DATA_BLOCK DB 49
TITLE =
VERSION : 0.1


  STRUCT
   Leiding : ARRAY  [0 .. 100 ] OF //Drukwaarde
   REAL  := 0.000000e+000;
  END_STRUCT ;
BEGIN
   Leiding[0] := 	1.138932E+00	;
Leiding[1] := 	1.155988E+00	;
Leiding[2] := 	1.173205E+00	;
Leiding[3] := 	1.190583E+00	;
Leiding[4] := 	1.208122E+00	;
Leiding[5] := 	1.225822E+00	;
Leiding[6] := 	1.243683E+00	;
Leiding[7] := 	1.261705E+00	;
Leiding[8] := 	1.279888E+00	;
Leiding[9] := 	1.298232E+00	;
Leiding[10] := 	1.316737E+00	;
Leiding[11] := 	1.335403E+00	;
Leiding[12] := 	1.354230E+00	;
Leiding[13] := 	1.373218E+00	;
Leiding[14] := 	1.392367E+00	;
Leiding[15] := 	1.411677E+00	;
Leiding[16] := 	1.431148E+00	;
Leiding[17] := 	1.450780E+00	;
Leiding[18] := 	1.470573E+00	;
Leiding[19] := 	1.490527E+00	;
Leiding[20] := 	1.510642E+00	;
Leiding[21] := 	1.530918E+00	;
Leiding[22] := 	1.551355E+00	;
Leiding[23] := 	1.571953E+00	;
Leiding[24] := 	1.592712E+00	;
Leiding[25] := 	1.613632E+00	;
Leiding[26] := 	1.634713E+00	;
Leiding[27] := 	1.655955E+00	;
Leiding[28] := 	1.677358E+00	;
Leiding[29] := 	1.698922E+00	;
Leiding[30] := 	1.720647E+00	;
Leiding[31] := 	1.742533E+00	;
Leiding[32] := 	1.764580E+00	;
Leiding[33] := 	1.786788E+00	;
Leiding[34] := 	1.809157E+00	;
Leiding[35] := 	1.831687E+00	;
Leiding[36] := 	1.854378E+00	;
Leiding[37] := 	1.877230E+00	;
Leiding[38] := 	1.900243E+00	;
Leiding[39] := 	1.923417E+00	;
Leiding[40] := 	1.946752E+00	;
Leiding[41] := 	1.970248E+00	;
Leiding[42] := 	1.993905E+00	;
Leiding[43] := 	2.017723E+00	;
Leiding[44] := 	2.041702E+00	;
Leiding[45] := 	2.065842E+00	;
Leiding[46] := 	2.090143E+00	;
Leiding[47] := 	2.114605E+00	;
Leiding[48] := 	2.139228E+00	;
Leiding[49] := 	2.164012E+00	;
Leiding[50] := 	2.188957E+00	;
Leiding[51] := 	2.214063E+00	;
Leiding[52] := 	2.239330E+00	;
Leiding[53] := 	2.264758E+00	;
Leiding[54] := 	2.290347E+00	;
Leiding[55] := 	2.316097E+00	;
Leiding[56] := 	2.342008E+00	;
Leiding[57] := 	2.368080E+00	;
Leiding[58] := 	2.394313E+00	;
Leiding[59] := 	2.420707E+00	;
Leiding[60] := 	2.447262E+00	;
Leiding[61] := 	2.473978E+00	;
Leiding[62] := 	2.500855E+00	;
Leiding[63] := 	2.527893E+00	;
Leiding[64] := 	2.555092E+00	;
Leiding[65] := 	2.582452E+00	;
Leiding[66] := 	2.609973E+00	;
Leiding[67] := 	2.637655E+00	;
Leiding[68] := 	2.665498E+00	;
Leiding[69] := 	2.693502E+00	;
Leiding[70] := 	2.721667E+00	;
Leiding[71] := 	2.749993E+00	;
Leiding[72] := 	2.778480E+00	;
Leiding[73] := 	2.807128E+00	;
Leiding[74] := 	2.835937E+00	;
Leiding[75] := 	2.864907E+00	;
Leiding[76] := 	2.894038E+00	;
Leiding[77] := 	2.923330E+00	;
Leiding[78] := 	2.952783E+00	;
Leiding[79] := 	2.982397E+00	;
Leiding[80] := 	3.012172E+00	;
Leiding[81] := 	3.042108E+00	;
Leiding[82] := 	3.072205E+00	;
Leiding[83] := 	3.102463E+00	;
Leiding[84] := 	3.132882E+00	;
Leiding[85] := 	3.163462E+00	;
Leiding[86] := 	3.194203E+00	;
Leiding[87] := 	3.225105E+00	;
Leiding[88] := 	3.256168E+00	;
Leiding[89] := 	3.287392E+00	;
Leiding[90] := 	3.318777E+00	;
Leiding[91] := 	3.350323E+00	;
Leiding[92] := 	3.382030E+00	;
Leiding[93] := 	3.413898E+00	;
Leiding[94] := 	3.445927E+00	;
Leiding[95] := 	3.478117E+00	;
Leiding[96] := 	3.510468E+00	;
Leiding[97] := 	3.542980E+00	;
Leiding[98] := 	3.575653E+00	;
Leiding[99] := 	3.608487E+00	;
Leiding[100] := 	3.641482E+00	;

END_DATA_BLOCK

